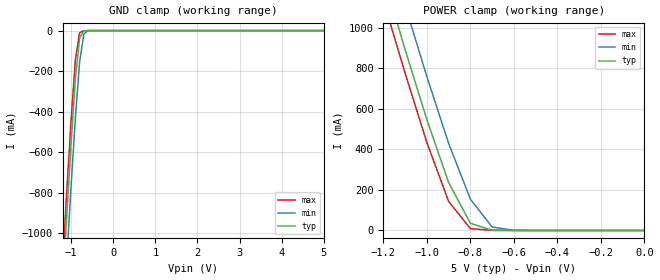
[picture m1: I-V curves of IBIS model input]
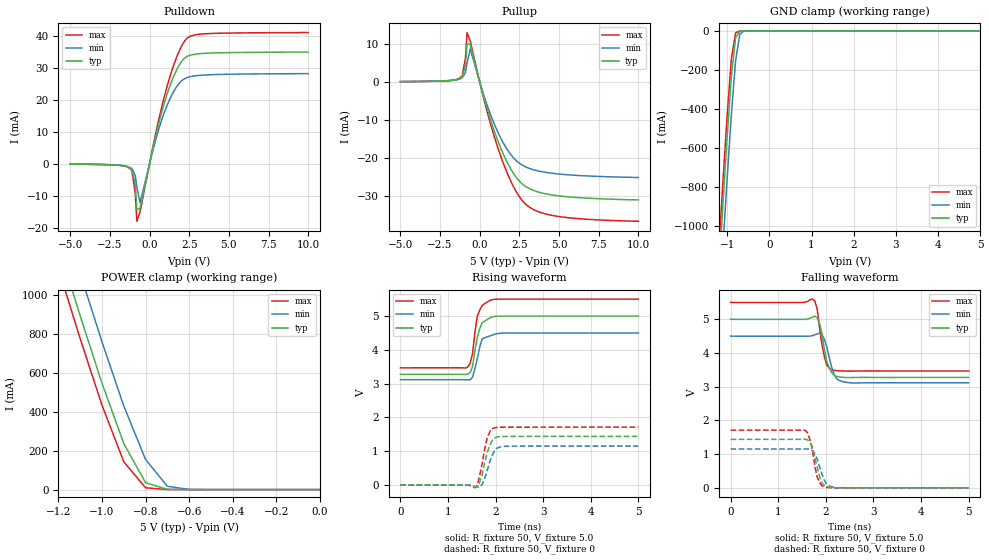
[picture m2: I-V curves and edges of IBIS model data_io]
| TSOP package &   Commercial  Operation
[IBIS Ver]   3.2
[Comment Char]   |_char
[File name]   as7c1024b_tsopc.ibs
[File Rev]   1.0
[Date]   Jun 7, 2004 4:26:03 PM
[Source]
Alliance Semiconductor Corporation
[Notes]
This model  is for TSOP package &
 Commercial  Operation
[Disclaimer]
Data is for modeling purpose only and is not guaranted.
This IBIS model is provided on an "AS IS" basis and Alliance Semiconductor makes
absolutely no warranty with respect to the information contained
herein.The entire risk as to quality and performance
is with the Customer. ACCORDINGLY, IN NO EVENT SHALL THE COMPANY BE
LIABLE FOR ANY DAMAGES, WHETHER IN CONTRACT OR TORT,INCLUDING ANY
LOST PROFITS OR OTHER INCIDENTAL, CONSEQUENTIAL, EXEMPLARY, OR
PUNITIVE DAMAGES ARISING OUT OF THE USE OR APPLICATION OF THE IBIS
model provided in this package.
[Copyright]
Alliance Semiconductor Corporation
| TSOP Package & Commercial Operation.
[Component]   AS7C1024B_TSOPC
Si_location Pin
Timing_location Pin
[Manufacturer]   Alliance Semiconductor Corporation
[Package]
R_pkg   226.75m   113.8m   339.7m
L_pkg   5.159nH   3.003nH   7.315nH
C_pkg   0.7210pF   0.51pF   0.932pF
[Pin] signal_name   model_name
1   A11   input
2   A9   input
3   A8   input
4   A13   input
5   NWE   input
6   CE2   input
7   A15   input
8   VSS   POWER
9   NC   NC
10   A16   input
11   A14   input
12   A12   input
13   A7   input
14   A6   input
15   A5   input
16   A4   input
17   A3   input
18   A2   input
19   A1   input
20   A0   input
21   IO0   data_io
22   IO1   data_io
23   IO2   data_io
24   GND   GND
25   IO3   data_io
26   IO4   data_io
27   IO5   data_io
28   IO6   data_io
29   IO7   data_io
30   NCE1   input
31   A10   input
32   NOE   input
| Models and submodels in the file (2): input (Input), data_io (I/O)
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[Model]   input
Model_type Input
Vinh=2.2V
Vinl=0.8V
C_comp   4pF   4pF   4pF
[Model Spec]
[Temperature Range] 25   70   0
[Voltage Range]   5.0   4.5   5.5
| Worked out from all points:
|   GND clamp passes 1 mA (typ) near -0.67 V on its own axis
|   POWER clamp passes 1 mA (typ) near -0.68 V on its own axis
[GND Clamp]
-5V       -16.01A    -16.21A    -15.91A
-1.2V     -1.253A    -1.472A    -1.135A
-1.1V     -892.6mA   -1.11A     -775.9mA
-1V       -547.3mA   -759.1mA   -435mA
-900mV    -237.4mA   -430.4mA   -144.1mA
-800mV    -36.26mA   -154.9mA   -10.33mA
-700mV    -1.383mA   -17.31mA   -546.7uA
-600mV    -81.45uA   -732.3uA   -58.64uA
5V        292.5pA    38.81uA    -1.719nA
[POWER Clamp]
-5V       16.01A     16.21A     15.9A
-1.2V     1.252A     1.471A     1.135A
-1.1V     891.7mA    1.109A     775mA
-1V       546.1mA    758.3mA    433.5mA
-900mV    236.6mA    429.1mA    142.8mA
-800mV    35.4mA     154.3mA    9.383mA
-700mV    1.248mA    17.09mA    442.2uA
-600mV    85.03uA    719uA      72.84uA
0V        292.5pA    1.265nA    178.1pA
[Model]   data_io
Model_type I/O
Enable Active-High
Polarity Non-Inverting
Vinh=2.2V
Vinl=0.8V
Vref=1.728V
Vmeas=1.5V
Rref=168
Cref=30pF
C_comp   4pF   4pF   4pF
[Temperature Range] 25   70   0
[Voltage Range]   5.0   4.5   5.5
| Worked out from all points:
|   slope of the pulldown table from 0 to 0.75 V, typ, clamps not added: 47.5 ohm
|   slope of the pullup table from 0 to 0.75 V, typ, clamps not added: 69.3 ohm
|   GND clamp passes 1 mA (typ) near -0.67 V on its own axis
|   POWER clamp passes 1 mA (typ) near -0.68 V on its own axis
|   falling waveform, R_fixture 50, V_fixture 5.0: 20-80 % time 149ps typ, 156ps min, 136ps max; typ from 5 V to 3.27 V
|   falling waveform, R_fixture 50, V_fixture 0: 20-80 % time 154ps typ, 170ps min, 138ps max; typ from 1.44 V to 0.003 V
|   rising waveform, R_fixture 50, V_fixture 5.0: 20-80 % time 148ps typ, 141ps min, 129ps max; typ from 3.27 V to 5 V
|   rising waveform, R_fixture 50, V_fixture 0: 20-80 % time 158ps typ, 165ps min, 145ps max; typ from 0 V to 1.44 V
[Pullup]
-5V       90uA       90uA       90uA
-1.2V     1.068mA    884uA      1.19mA
-1.1V     1.45mA     1.138mA    1.681mA
-900mV    4.251mA    2.482mA    6.248mA
-800mV    9.897mA    4.922mA    12.98mA
-600mV    9.913mA    8.667mA    10.8mA
300mV     -4.636mA   -4.026mA   -5.101mA
1.1V      -15.02mA   -12.81mA   -16.77mA
2V        -23.2mA    -19.31mA   -26.44mA
2.7V      -26.89mA   -21.92mA   -31.3mA
4.7V      -29.79mA   -24.08mA   -35.19mA
10V       -31.02mA   -25.12mA   -36.64mA
[Pulldown]
-5V       -120uA     -120uA     -120uA
-1.2V     -1.484mA   -1.217mA   -1.62mA
-1.1V     -2.045mA   -1.613mA   -2.332mA
-900mV    -6.312mA   -3.654mA   -9.329mA
-800mV    -14.39mA   -7.31mA    -18.01mA
-600mV    -13.97mA   -12.18mA   -15.07mA
300mV     6.815mA    5.893mA    7.407mA
1.1V      21.68mA    18.21mA    24.11mA
1.7V      29.3mA     24.06mA    33.26mA
2.3V      33.43mA    26.86mA    38.99mA
3.6V      34.6mA     27.82mA    40.72mA
10V       34.96mA    28.22mA    41.07mA
[GND Clamp]
-5V       -16.01A    -16.21A    -15.91A
-1.2V     -1.253A    -1.472A    -1.135A
-1.1V     -892.6mA   -1.11A     -775.9mA
-1V       -547.3mA   -759.1mA   -435mA
-900mV    -237.4mA   -430.4mA   -144.1mA
-800mV    -36.26mA   -154.9mA   -10.33mA
-700mV    -1.383mA   -17.31mA   -546.7uA
-600mV    -81.45uA   -732.3uA   -58.64uA
5V        292.5pA    38.81uA    -1.719nA
[POWER Clamp]
-5V       16.01A     16.21A     15.9A
-1.2V     1.252A     1.471A     1.135A
-1.1V     891.7mA    1.109A     775mA
-1V       546.1mA    758.3mA    433.5mA
-900mV    236.6mA    429.1mA    142.8mA
-800mV    35.4mA     154.3mA    9.383mA
-700mV    1.248mA    17.09mA    442.2uA
-600mV    85.03uA    719uA      72.84uA
0V        292.5pA    1.265nA    178.1pA
[Falling Waveform]
R_fixture=50
V_fixture=5.0
V_fixture_min=4.5
V_fixture_max=5.5
0s        5V         4.5V       5.5V
1.717ns   5.056V     4.511V     5.596V
1.768ns   5.091V     4.538V     5.547V
1.818ns   5.05V      4.563V     5.314V
1.919ns   4.586V     4.546V     4.262V
2.02ns    3.751V     4.193V     3.644V
2.121ns   3.424V     3.592V     3.504V
2.222ns   3.305V     3.241V     3.476V
2.525ns   3.272V     3.114V     3.464V
5ns       3.274V     3.117V     3.466V
[Falling Waveform]
R_fixture=50
V_fixture=0
V_fixture_min=0
V_fixture_max=0
0s        1.438V     1.152V     1.712V
1.566ns   1.443V     1.155V     1.708V
1.616ns   1.423V     1.155V     1.637V
1.667ns   1.358V     1.151V     1.432V
1.717ns   1.215V     1.114V     1.139V
1.818ns   629.7mV    864.5mV    324.8mV
1.919ns   140.9mV    413.9mV    64.43mV
2.02ns    35.44mV    104mV      15.86mV
2.323ns   3.368mV    5.371mV    2.989mV
5ns       2.726mV    2.673mV    2.893mV
[Rising Waveform]
R_fixture=50
V_fixture=5.0
V_fixture_min=4.5
V_fixture_max=5.5
0s        3.275V     3.117V     3.466V
1.414ns   3.28V      3.114V     3.487V
1.465ns   3.327V     3.112V     3.603V
1.515ns   3.5V       3.188V     3.875V
1.566ns   3.969V     3.448V     4.507V
1.616ns   4.368V     3.735V     4.994V
1.717ns   4.8V       4.319V     5.307V
1.919ns   4.966V     4.428V     5.478V
2.222ns   4.997V     4.496V     5.496V
5ns       4.997V     4.497V     5.496V
[Rising Waveform]
R_fixture=50
V_fixture=0
V_fixture_min=0
V_fixture_max=0
0s        0V         502.4nV    0V
1.566ns   -66.94mV   -41.15mV   -80.71mV
1.616ns   -49.61mV   -59.63mV   -10.77mV
1.667ns   92.94mV    -49.64mV   289.3mV
1.717ns   301.9mV    16.03mV    627.2mV
1.818ns   931.5mV    393.1mV    1.367V
1.919ns   1.3V       859mV      1.667V
1.97ns    1.375V     993.4mV    1.69V
2.222ns   1.439V     1.15V      1.712V
5ns       1.44V      1.153V     1.714V
[Ramp]
R_load=50
dV/dt_r   8.639E-1/1.562E-10   6.920E-1/1.636E-10   1.028E+0/1.437E-10
dV/dt_f   1.035E+0/1.438E-10   8.299E-1/1.531E-10   1.220E+0/1.350E-10
|[End   data_io
